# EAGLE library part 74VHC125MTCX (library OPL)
Quad Buffer/Line Driver;3-state
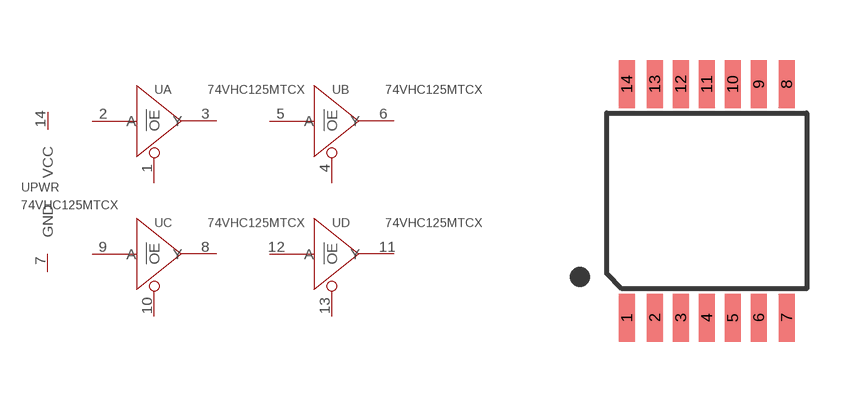
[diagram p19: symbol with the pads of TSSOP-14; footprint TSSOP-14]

Designator prefix U; gates A=BUFFER PWR=VCC-GND-1 B=BUFFER C=BUFFER D=BUFFER

## 74VHC125MTCXHC-310050042, 74VHC125MTCXHCT-310050042  [TSSOP-14]
1  A:!OE
2  A:A
3  A:Y
4  B:!OE
5  B:A
6  B:Y
7  PWR:GND  sup
8  C:Y
9  C:A
10  C:!OE
11  D:Y
12  D:A
13  D:!OE
14  PWR:VCC  sup

## Footprint TSSOP-14 (pad centres in mm)
smd 0.4 x 1.2: 1 -2,-2.925; 2 -1.3,-2.925; 3 -0.65,-2.925; 4 0,-2.925; 5 0.65,-2.925; 6 1.3,-2.925; 7 2,-2.925; 8 2,2.925; 9 1.3,2.925; 10 0.65,2.925; 11 0,2.925; 12 -0.65,2.925; 13 -1.3,2.925; 14 -2,2.925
